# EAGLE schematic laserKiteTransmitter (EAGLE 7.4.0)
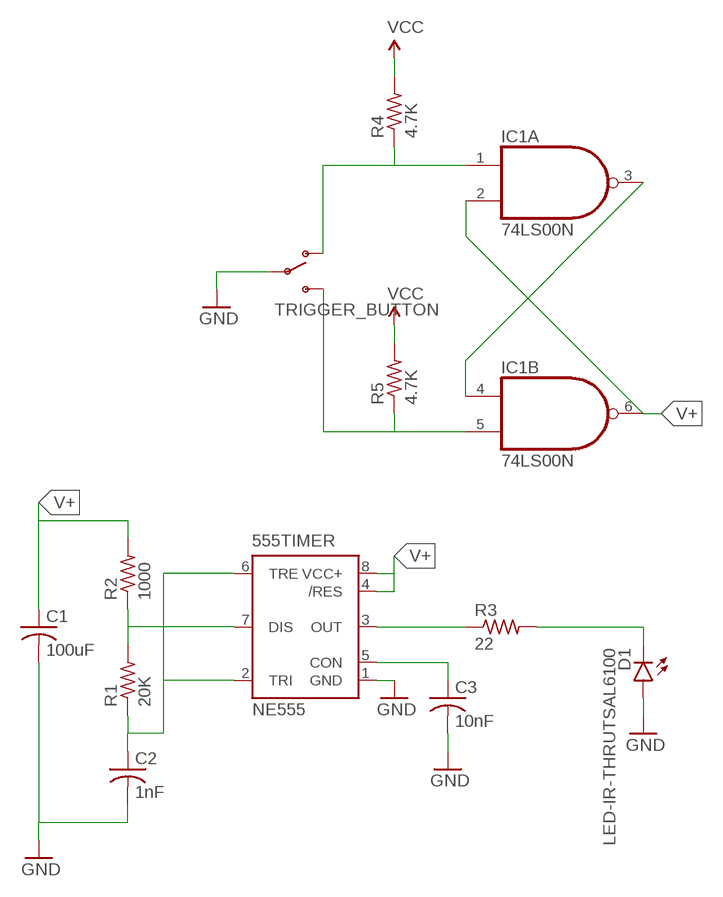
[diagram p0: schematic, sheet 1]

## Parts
555TIMER  NE555  [DIL-08]
C1  100uF  C-US025-050X050  [C025-050X050]
C2  1nF  C-US025-025X050  [C025-025X050]
C3  10nF  C-US025-025X050  [C025-025X050]
D1  LED-IR-THRUTSAL6100  [LED5MM]
IC1  74LS00N  [DIL14]
R1  20K  R-US_0207/2V  [0207/2V]
R2  1000  R-US_0207/2V  [0207/2V]
R3  22  R-US_0207/9  [0207/9]
R4  4.7K  R-US_0207/2V  [0207/2V]
R5  4.7K  R-US_0207/2V  [0207/2V]
TRIGGER_BUTTON  SWITCH-SPDTKIT  [SWITCH-SPDT_KIT]

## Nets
GND: 555TIMER.1(GND) C1.2 C2.2 C3.2 D1.A TRIGGER_BUTTON.2(P)
N$1: 555TIMER.7(DIS) R1.2 R2.1
N$2: IC1.3(A:O) IC1.4(B:I0)
N$3: IC1.1(A:I0) R4.1 TRIGGER_BUTTON.1(O)
N$4: IC1.5(B:I1) R5.1 TRIGGER_BUTTON.3(S)
N$5: 555TIMER.2(TRI) 555TIMER.6(TRE) C2.1 R1.1
N$6: 555TIMER.5(CON) C3.1
N$7: 555TIMER.3(OUT) R3.1
N$8: D1.K(C) R3.2
V+: 555TIMER.4(/RES) 555TIMER.8(VCC+) C1.1 IC1.2(A:I1) IC1.6(B:O) R2.2
VCC: R4.2 R5.2
Unconnected: IC1.8(C:O) IC1.9(C:I0) IC1.10(C:I1) IC1.11(D:O) IC1.12(D:I0) IC1.13(D:I1)

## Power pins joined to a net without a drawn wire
GND: IC1.7(P:GND)
VCC: IC1.14(P:VCC)

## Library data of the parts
555TIMER = st-microelectronics:NE555: General purpose bipolar Timer; MF: Arrow Electronics; MPN: NE555N; OC_FARNELL: 1467742; OC_NEWARK: 89K1486
C1-C3 = adafruit:C-US: CAPACITOR, American symbol
D1 = SparkFun-LED:LED-IR-THRU; PROD_ID: DIO-12058
IC1 = 74xx-us:74*00: Quad 2-input NAND gate
R1-R5 = adafruit:R-US_: RESISTOR, American symbol
TRIGGER_BUTTON = SparkFun-Electromechanical:SWITCH-SPDT: SPDT Switch Simple slide switch, Spark Fun Electronics SKU : COM-00102 DPDT SMT slide switch, AYZ0202, SWCH-08179; PROD_ID: SWCH-08261

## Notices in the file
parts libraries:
SparkFun-LED: Licensing: Creative Commons ShareAlike 4.0 International - https://creativecommons.org/licenses/by-sa/4.0
